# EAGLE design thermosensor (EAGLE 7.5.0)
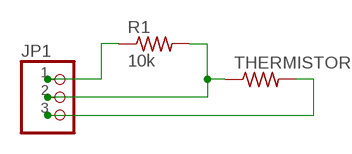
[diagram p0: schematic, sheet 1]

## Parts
JP1  PINHD-1X3  [1X03]
R1  10k  RES-US1206FAB  [R1206FAB]
THERMISTOR  RES-US1206FAB  [R1206FAB]

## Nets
N$1: JP1.1 R1.1
N$2: JP1.3 THERMISTOR.2
N$3: JP1.2 R1.2 THERMISTOR.1

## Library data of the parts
JP1 = pinhead:PINHD-1X3: PIN HEADER
R1 THERMISTOR = fab:RES-US: Resistor (US Symbol)

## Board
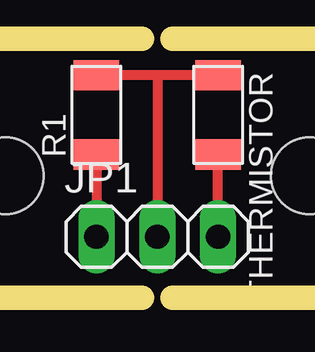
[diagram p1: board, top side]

No outline drawn. Coordinates in mm, seen from the top.
Copper layers (1*16): Top 0.035mm / dielectric 1.5mm / Bottom 0.035mm
Design rules "default": minimum track width 10mil, minimum drill 24mil, track to track 8mil, track to pad 8mil, pad to pad 8mil, via to via 8mil, smd to smd 8mil, copper to edge 40mil, drill to drill 8mil, minimum pad ring 10mil, minimum via ring 8mil, stop-mask expansion 4mil, vias tented up to drill 0mil, thermal gap 10mil
Holes 3.2 mm at 30.48,24.13 17.78,24.13
Milling: 10 lines

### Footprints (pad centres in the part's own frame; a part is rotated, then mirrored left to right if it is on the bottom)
1X03 = drill 1.016 long: 1 -2.54,0; 2 0,0; 3 2.54,0
R1206FAB = smd 1.27 x 1.905: 1 -1.651,0; 2 1.651,0

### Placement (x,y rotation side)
JP1  24.13,21.59 0 top
R1  21.59,26.67 90 top
THERMISTOR  26.67,26.67 270 top

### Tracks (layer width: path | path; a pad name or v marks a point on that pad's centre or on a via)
N$1
  Top 0.406: R1.1 JP1.1
N$2
  Top 0.406: JP1.3 THERMISTOR.2
N$3
  Top 0.406: R1.2 THERMISTOR.1 24.13,28.32 JP1.2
